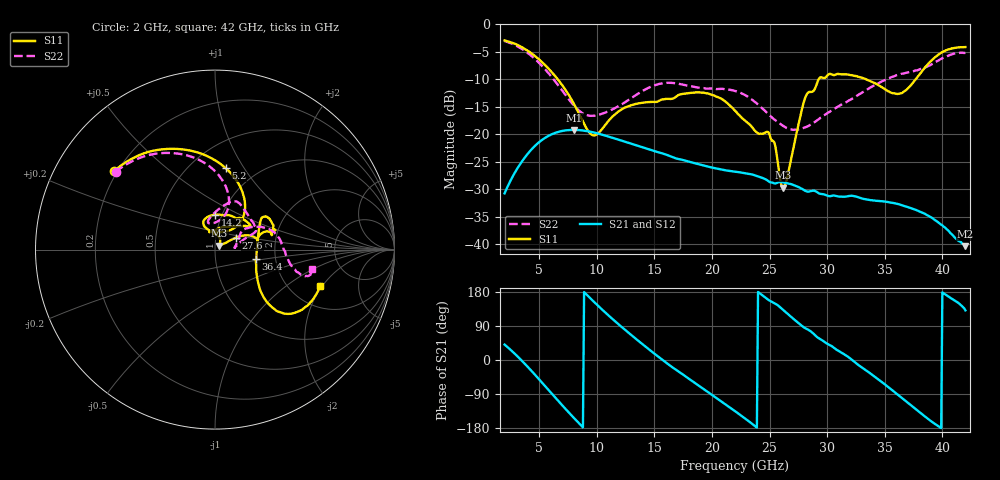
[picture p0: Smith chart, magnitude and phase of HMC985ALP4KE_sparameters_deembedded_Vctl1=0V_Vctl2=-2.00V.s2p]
!s2p File: Measurements: S11, S21, S12, S22
# GHz S dB R 50.0
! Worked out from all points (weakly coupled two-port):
!   401 points, 2 GHz to 42 GHz, reference 50 ohm
!   highest |S21| = -19.20 dB at 8 GHz (marker M1); lowest = -40.4 dB at 42 GHz (marker M2)
!   lowest |S11| = -29.7 dB at 26.2 GHz (marker M3), VSWR 1.07, Z = 52.3 + j2.39 ohm
!   |S11| at or under -10 dB: 6.608 GHz to 29.27 GHz (22.66 GHz wide, 126 % of centre); 33.36 GHz to 37.7 GHz (4.333 GHz wide, 12.2 % of centre)
!   |S22| runs from -19.2 to -3.1 dB; largest |S21 - S12| = 0.00017
!   S11 on the Smith chart (normalised r, x): 2 GHz: 0.19, +0.33; 5.2 GHz: 0.73, +0.83; 14.2 GHz: 0.93, +0.38; 27.6 GHz: 1.25, +0.17; 36.4 GHz: 1.58, -0.18; 42 GHz: 2.90, -1.91
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2  -2.95 142.0  -30.76 40.6  -30.76 40.6  -3.06 142.0
3.6  -4.31 112.8  -24.67 -5.1  -24.67 -5.1  -4.64 113.6
5.2  -6.80 82.4  -21.11 -58.0  -21.12 -58.0  -7.47 88.2
8  -14.40 47.1  -19.20 -152.4  -19.21 -152.5  -14.74 76.3
8.7  -17.30 52.2  -19.30 -174.6  -19.30 -174.6  -16.10 85.1
9.9  -20.16 89.8  -19.77 149.2  -19.77 149.2  -16.59 100.8
12.1  -15.57 113.0  -21.13 88.8  -21.13 88.8  -14.64 97.2
14.2  -14.21 89.7  -22.50 36.0  -22.50 36.0  -11.86 77.6
15.4  -13.94 73.1  -23.31 7.7  -23.32 7.6  -10.86 69.7
19.3  -12.45 34.3  -25.71 -77.1  -25.71 -77.1  -11.62 40.9
22  -15.69 52.3  -26.81 -134.9  -26.82 -134.9  -12.13 23.9
25  -20.07 98.5  -28.68 156.9  -28.69 156.9  -16.56 16.7
26.2  -29.72 44.2  -28.76 131.3  -28.76 131.3  -18.52 8.8
27.6  -17.40 29.6  -29.69 95.0  -29.70 95.1  -19.05 6.8
28.1  -13.32 20.9  -30.29 83.9  -30.30 83.9  -18.77 9.8
28.7  -12.29 13.0  -30.28 72.5  -30.28 72.4  -18.07 15.0
31  -9.06 23.3  -31.33 24.0  -31.34 24.0  -14.88 34.2
33.3  -9.94 34.2  -31.81 -25.8  -31.84 -25.8  -12.12 30.4
35.4  -12.27 12.2  -32.39 -73.7  -32.38 -73.7  -9.80 20.2
36.4  -12.58 -13.0  -32.86 -98.1  -32.87 -98.1  -9.04 13.9
39.5  -5.81 -43.4  -35.81 -171.5  -35.83 -171.4  -6.75 -14.0
42  -4.15 -19.0  -40.35 131.1  -40.33 131.0  -5.20 -11.2
